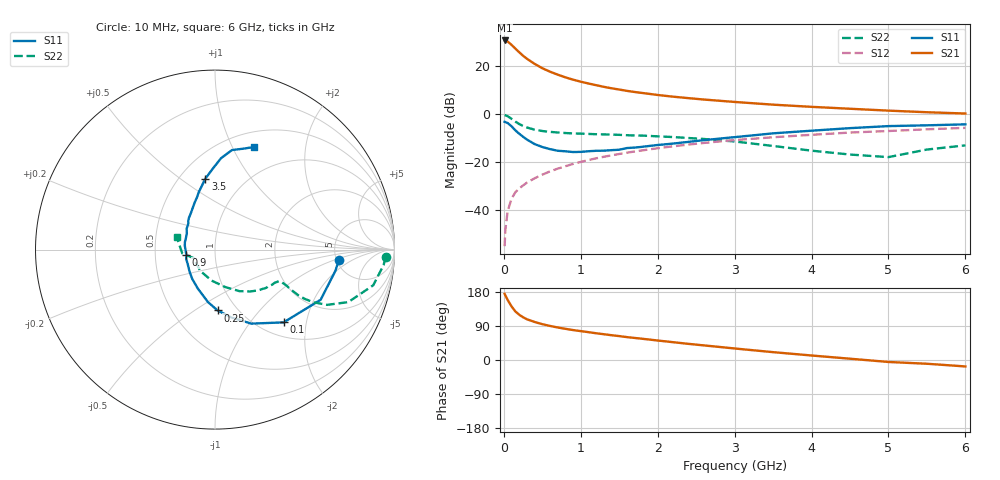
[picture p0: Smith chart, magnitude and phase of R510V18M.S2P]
! SIEMENS Small Signal Semiconductors
! BFR183
! Si NPN RF Bipolar Junction Transistor in SOT23
! VCE = 10 V  IC = 18 mA
! Common Emitter S-Parameters:  May  1996
# GHz  S  MA  R  50
!  f  S11  S21  S12  S22
! GHz  MAG  ANG  MAG  ANG  MAG  ANG  MAG  ANG
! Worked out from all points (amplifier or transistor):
!   36 points, 10 MHz to 6 GHz, reference 50 ohm
!   highest |S21| = 30.6 dB at 10 MHz (marker M1)
!   |S21| within 3 dB of that: start of sweep to 137.6 MHz
!   unconditionally stable (mu >= 1): 672.6 MHz to 2.625 GHz
!   at 250 MHz: K = 0.75, MSG = 27.0 dB, |S12| = -29.7 dB
!   at 1.4 GHz: K = 1.04, MAG = 12.7 dB, |S12| = -17.2 dB
!   at 6 GHz: K = 0.90, MSG = 3.0 dB, |S12| = -5.7 dB
!   S11 on the Smith chart (normalised r, x): 10 MHz: 5.21, -1.21; 100 MHz: 1.26, -1.48; 250 MHz: 0.81, -0.62; 900 MHz: 0.72, -0.04; 3.5 GHz: 0.66, +0.62; 6 GHz: 0.67, +1.22
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0.01  0.6923 -5.0  33.91 174.6  0.0018 69.7  0.9519 -2.4
0.02  0.6809 -10.1  33.67 170.3  0.004 75.2  0.9434 -5.2
0.05  0.6515 -25.4  32.15 158.3  0.0097 77.3  0.9038 -12.7
0.1  0.5572 -46.7  27.46 141.5  0.0174 69.8  0.7982 -21.5
0.15  0.4592 -63.9  22.96 128.1  0.0238 67.6  0.6972 -26.2
0.2  0.3901 -76.2  19.25 119.4  0.0286 66.7  0.6217 -28.2
0.25  0.3391 -87.6  16.31 112.8  0.0329 65.7  0.5668 -28.8
0.3  0.2956 -97.5  14.14 107.5  0.0377 66.9  0.5267 -28.7
0.4  0.238 -113.5  11.07 100.4  0.0464 68.3  0.4747 -27.7
0.5  0.2072 -127.6  8.984 94.5  0.0551 68.9  0.4449 -26.7
0.6  0.1869 -139.6  7.611 89.9  0.0645 69.4  0.4273 -26.3
0.7  0.173 -150.9  6.605 85.8  0.0735 69.6  0.4149 -26.2
0.9  0.1626 -169.7  5.193 79.0  0.0923 68.7  0.3965 -26.4
1.1  0.1691 173.5  4.322 73.5  0.1108 67.9  0.3872 -28.0
1.3  0.1736 159.9  3.684 68.0  0.1298 66.4  0.3783 -29.8
1.6  0.197 143.2  3.04 60.4  0.1577 63.8  0.364 -33.5
2.2  0.2439 123.4  2.301 47.0  0.2142 57.9  0.3335 -42.7
3.5  0.3983 97.8  1.57 20.7  0.3301 42.1  0.2176 -74.2
4.5  0.5106 86.2  1.291 3.4  0.4134 30.0  0.1443 -125.1
5  0.5627 80.3  1.18 -5.2  0.4451 22.8  0.1277 -158.1
5.5  0.5845 74.2  1.093 -9.9  0.4832 18.8  0.1834 -173.3
6  0.6126 69.0  1.027 -17.0  0.5173 11.6  0.2238 162.2
